| IBIS file k65_180_169wlcsp_derated.ibs generated by Daphne version: 2015.01.22
[IBIS Ver]   4.2
[Comment Char]   |_char
[File Name]   k65_180_169wlcsp_derated.ibs
[File Rev]   1.0
[Date]   Mon Feb  9 00:49:59 2015
[Source]   FSL Viper 2015.01.22
[Notes]
[Disclaimer] IMPORTANT NOTICE
  This information is provided on an AS IS basis and without warranty.
  IN NO EVENT SHALL Freescale BE LIABLE FOR INCIDENTAL OR CONSEQUENTIAL
  DAMAGES ARISING FROM USE OF THIS INFORMATION. THIS DISCLAIMER OF
  WARRANTY EXTENDS TO THE USER OF THE INFORMATION, AND TO THEIR CUSTOMERS
  OR USERS OF PRODUCTS  AND IS IN LIEU OF ALL WARRANTIES WHETHER EXPRESS,
  IMPLIED, OR STATUTORY, INCLUDING IMPLIED WARRANTIES OF MERCHANTABILITY
  OR FITNESS FOR PARTICULAR PURPOSE.
  Freescale does not represent or warrant that the information furnished
  hereunder is free of infringement of any third party patents,
  copyrights, trade secrets, or other intellectual property rights.
  Freescale does not represent or warrant that the information is free of
  defect, or that it meets any particular standard, requirements or need
  of the user of the infomation or their customers.
  Freescale reserves the right to change the information in this file
  without notice.
   http://www.freescale.com
[Copyright]   (C) Copyright Freescale 2004 - 2015, All Rights Reserved.
|   k65_169wlcsp
[Component]   k65_169wlcsp
[Manufacturer]   FREESCALE
[Package]
| variable   typ   min   max
R_pkg   0.15383   6.1113e-3   0.52143
L_pkg   5.764e-10   2.255e-11   1.965e-9
C_pkg   5.451e-13   3.559e-13   3.23e-12
[Pin] signal_name   model_name   R_pin   L_pin   C_pin
A1   PTC4   p_io_fast_hd_84u3v_6m   0.023732  8.85e-11  3.766e-13
A2   PTC9   p_io_fast_84u3v_6m   0.018375  6.862e-11 3.613e-13
A3   PTC13   p_io_fast_84u3v_6m   0.018129  6.765e-11 3.623e-13
A4   PTC15   p_io_fast_84u3v_6m   0.026124  9.752e-11 3.789e-13
A5   PTC16   p_io_fast_84u3v_6m   0.022637  8.435e-11 3.688e-13
A6   PTC24   p_io_fast_84u3v_6m   0.022119  8.262e-11 3.667e-13
A7   PTC27   p_io_fast_84u3v_6m   0.013327  4.926e-11 3.772e-13
A8   PTD1   p_io_fast_84u3v_6m   0.020798  7.767e-11 3.64e-13
A9   PTD5   p_io_fast_hd_84u3v_6m   0.024872  9.264e-11 3.787e-13
A10   PTD7   p_io_fast_hd_84u3v_6m   0.056991  2.143e-10 3.903e-13
A11   PTD10   p_io_fast_84u3v_6m   0.038132  1.422e-10 3.951e-13
A12   PTD13   p_io_fast_84u3v_6m   0.030801  1.148e-10 3.876e-13
A13   PTE1   p_io_fast_84u3v_6m   0.028905  9.982e-11 3.814e-13
B1   PTC3   p_io_fast_hd_84u3v_6m   0.02893   1.024e-10 3.939e-13
B2   PTC5   p_io_fast_84u3v_6m   0.11805   4.455e-10 4.334e-13
B3   PTC10   p_io_fast_84u3v_6m   0.083692  3.154e-10 4.487e-13
B4   PTC14   p_io_fast_84u3v_6m   0.076299  2.875e-10 4.432e-13
B5   PTC17   p_io_fast_84u3v_6m   0.081732  3.078e-10 4.521e-13
B6   PTC19   p_io_fast_84u3v_6m   0.07776   2.928e-10 4.431e-13
B7   PTC28   p_io_fast_84u3v_6m   0.095167  3.59e-10  4.232e-13
B8   PTD2   p_io_fast_84u3v_6m   0.098354  3.71e-10  4.199e-13
B9   PTD6   p_io_fast_hd_84u3v_6m   0.11099   4.135e-10 4.308e-13
B10   PTD9   p_io_fast_84u3v_6m   0.10858   4.097e-10 4.919e-13
B11   PTD14   p_io_fast_84u3v_6m   0.15851   5.985e-10 4.673e-13
B12   PTE2   p_io_fast_84u3v_6m   0.093952  3.43e-10  4.731e-13
B13   PTE3   p_io_fast_84u3v_6m   0.040384  1.405e-10 4.018e-13
C1   PTC0   p_io_fast_84u3v_6m   0.045045  1.537e-10 3.845e-13
C2   PTC1   p_io_fast_84u3v_6m   0.09143   3.347e-10 4.691e-13
C3   PTC6   p_io_fast_84u3v_6m   0.21207   8.018e-10 5.038e-13
C4   PTC8   p_io_fast_84u3v_6m   0.24924   9.43e-10  5.323e-13
C5   PTC12   p_io_fast_84u3v_6m   0.19362   7.319e-10 6.054e-13
C6   PTC18   p_io_fast_84u3v_6m   0.13228   4.993e-10 5.174e-13
C7   PTC29   p_io_fast_84u3v_6m   0.17049   6.443e-10 4.713e-13
C8   PTD3   p_io_fast_84u3v_6m   0.1722   6.501e-10 4.686e-13
C9   PTD8   p_io_fast_84u3v_6m   0.18018   6.805e-10 5.792e-13
C10   PTD12   p_io_fast_84u3v_6m   0.23589   8.918e-10 5.241e-13
C11   PTE0   p_io_fast_84u3v_6m   0.18527   6.998e-10 5.94e-13
C12   PTE4   p_io_fast_84u3v_6m   0.085377  3.141e-10 4.617e-13
C13   PTE6   p_io_fast_84u3v_6m   0.024732  8.58e-11  3.806e-13
D1   PTB21   p_io_fast_84u3v_6m   0.042455  1.491e-10 4.054e-13
D2   PTB22   p_io_fast_84u3v_6m   0.095598  3.503e-10 4.76e-13
D3   PTB23   p_io_fast_84u3v_6m   0.15005   5.554e-10 5.454e-13
D4   PTC2   p_io_fast_84u3v_6m   0.22558   8.431e-10 6.474e-13
D5   PTC7   p_io_fast_84u3v_6m   0.36302   1.373e-9  6.151e-13
D6   PTC11   p_io_fast_84u3v_6m   0.28083   1.062e-9  7.192e-13
D7   PTC25   p_io_fast_84u3v_6m   0.24737   9.352e-10 5.244e-13
D8   PTD0   p_io_fast_84u3v_6m   0.24069   9.1e-10   5.199e-13
D9   PTD11   p_io_fast_84u3v_6m   0.32905   1.244e-9  5.966e-13
D10   PTD15   p_io_fast_84u3v_6m   0.25457   9.624e-10 6.869e-13
D11   PTE5   p_io_fast_84u3v_6m   0.1582   5.936e-10 5.659e-13
D12   PTE8   p_io_fast_84u3v_6m   0.080106  2.969e-10 4.574e-13
D13   PTE9   p_io_fast_84u3v_6m   0.02551   8.823e-11 3.825e-13
E1   PTB16   p_io_fast_84u3v_6m   0.039133  1.335e-10 6.001e-13
E2   PTB17   p_io_fast_84u3v_6m   0.11944   4.359e-10 4.4e-13
E3   PTB18   p_io_fast_84u3v_6m   0.19455   7.186e-10 4.928e-13
E4   PTB19   p_io_fast_84u3v_6m   0.27322   1.019e-9  5.501e-13
E5   PTB20   p_io_fast_84u3v_6m   0.35239   1.319e-9  6.063e-13
E6   VDD   POWER   NA   NA   NA
E7   VDD   POWER   NA   NA   NA
E8   PTC26   p_io_fast_84u3v_6m   0.3454   1.307e-9  5.975e-13
E9   VDD   POWER   NA   NA   NA
E10   PTE7   p_io_fast_84u3v_6m   0.21217   7.942e-10 6.304e-13
E11   PTE11   p_io_fast_84u3v_6m   0.13874   5.131e-10 5.227e-13
E12   PTE12   p_io_fast_84u3v_6m   0.081914  3.035e-10 4.562e-13
E13   VDD   POWER   NA   NA   NA
F1   PTB15   p_io_fast_84u3v_6m   0.037248  1.296e-10 5.892e-13
F2   PTB14   p_io_fast_84u3v_6m   0.1199   4.397e-10 4.397e-13
F3   PTB13   p_io_fast_84u3v_6m   0.18578   6.906e-10 4.872e-13
F4   PTB12   p_io_fast_84u3v_6m   0.25216   9.457e-10 5.394e-13
F5   PTB11   p_io_fast_84u3v_6m   0.31655   1.193e-9  5.865e-13
F6   VSS   GND   NA   NA   NA
F7   VSS   GND   NA   NA   NA
F8   PTD4   p_io_fast_hd_84u3v_6m   0.38395   1.452e-9  6.24e-13
F9   VDD   POWER   NA   NA   NA
F10   PTE10   p_io_fast_84u3v_6m   0.23213   8.667e-10 6.526e-13
F11   PTE17   p_io_fast_84u3v_6m   0.18215   6.744e-10 4.906e-13
F12   PTE19   p_io_fast_84u3v_6m   0.12637   4.625e-10 4.553e-13
F13   VSS   GND   NA   NA   NA
G1   PTB10   p_io_fast_84u3v_6m   0.025215  8.729e-11 3.82e-13
G2   PTB9   p_io_fast_84u3v_6m   0.11037   3.994e-10 4.374e-13
G3   PTB8   p_io_fast_84u3v_6m   0.17439   6.504e-10 4.747e-13
G4   PTB7   p_io_fast_84u3v_6m   0.24603   9.208e-10 5.301e-13
G5   PTB6   p_io_fast_84u3v_6m   0.32096   1.199e-9  5.843e-13
G6   VDD   POWER   NA   NA   NA
G7   VSS   GND   NA   NA   NA
G8   VSS   GND   NA   NA   NA
G9   PTE16   p_io_fast_84u3v_6m   0.36509   1.369e-9  6.196e-13
G10   PTE18   p_io_fast_84u3v_6m   0.28872   1.074e-9  5.683e-13
G11   VREGOUT   POWER   0.28285   1.07e-9   6.103e-13
G12   VREGIN0   POWER   0.11913   4.476e-10 5.637e-13
G13   USB0DP   NC   0.040105  1.411e-10 4.143e-13
H1   PTB5   p_io_fast_84u3v_6m   0.02475   8.564e-11 3.808e-13
H2   PTB4   p_io_fast_84u3v_6m   0.082285  3.039e-10 4.551e-13
H3   PTB3   p_io_fast_84u3v_6m   0.1553   5.764e-10 5.545e-13
H4   PTB0   p_io_fast_hd_84u3v_6m   0.22249   8.274e-10 6.597e-13
H5   PTA31   p_io_fast_84u3v_6m   0.28767   1.078e-9  7.367e-13
H6   VSS   GND   NA   NA   NA
H7   VSS   GND   NA   NA   NA
H8   TAMPER6   p_io_84u3v_6m   0.40121   1.518e-9  6.321e-13
H9   TAMPER2   p_io_84u3v_6m   0.42606   1.613e-9  6.532e-13
H10   TAMPER1   p_io_84u3v_6m   0.43051   1.629e-9  6.596e-13
H11   ADC1SE16_CMP2IN2_ADC0SE22   NC   0.52143   1.965e-9  7.296e-13
H12   VREGIN1   POWER   0.081939  3.085e-10 5.05e-13
H13   USB0DM   NC   0.042727  1.498e-10 4.137e-13
J1   PTB2   p_io_fast_84u3v_6m   0.036541  1.276e-10 3.982e-13
J2   PTB1   p_io_fast_hd_84u3v_6m   0.090111  3.314e-10 6.961e-13
J3   PTA26   p_io_fast_84u3v_6m   0.30189   1.127e-9  5.72e-13
J4   PTA25   p_io_fast_84u3v_6m   0.36496   1.363e-9  6.172e-13
J5   PTA9   p_io_fast_84u3v_6m   0.36508   1.381e-9  6.152e-13
J6   PTA3   p_io_fast_84u3v_6m   0.31893   1.206e-9  5.775e-13
J7   PTE27   p_io_fast_84u3v_6m   0.30618   1.158e-9  5.656e-13
J8   TAMPER7   p_io_84u3v_6m   0.32279   1.223e-9  5.759e-13
J9   TAMPER3   p_io_84u3v_6m   0.34626   1.31e-9   5.974e-13
J10   TAMPER0_RTCWAKEUP   p_io_84u3v_6m   0.37467   1.418e-9  6.188e-13
J11   ADC1DP1   NC   0.18235   6.796e-10 6.053e-13
J12   USB1VSS   GND   NA   NA   NA
J13   USB1DP   NC   0.035762  1.286e-10 4.048e-13
K1   PTA30   p_io_fast_84u3v_6m   0.044808  1.573e-10 4.101e-13
K2   PTA29   p_io_fast_84u3v_6m   0.097255  3.561e-10 4.771e-13
K3   PTA24   p_io_fast_84u3v_6m   0.26349   9.776e-10 5.455e-13
K4   PTA16   p_io_fast_84u3v_6m   0.28673   1.085e-9  5.539e-13
K5   PTA10   p_io_fast_84u3v_6m   0.30667   1.16e-9   5.738e-13
K6   PTA4   p_io_flt_84u3v_6m   0.2545   9.6e-10   5.382e-13
K7   PTE28   p_io_fast_84u3v_6m   0.24086   9.108e-10 5.207e-13
K8   VDD   POWER   NA   NA   NA
K9   TAMPER5   p_io_84u3v_6m   0.19261   7.28e-10  6.086e-13
K10   ADC0SE16_CMP1IN2_ADC0SE21   NC   0.35901   1.358e-9  6.097e-13
K11   ADC1DM1   NC   0.18943   7.059e-10 6.096e-13
K12   USB1VBUS   POWER   0.079962  2.996e-10 5.011e-13
K13   USB1DM   NC   0.033877  1.207e-10 4.021e-13
L1   PTA28   p_io_fast_84u3v_6m   0.032314  1.102e-10 3.958e-13
L2   PTA27   p_io_fast_84u3v_6m   0.11465   4.175e-10 4.36e-13
L3   PTA17   p_io_fast_84u3v_6m   0.2195   8.299e-10 5.116e-13
L4   PTA15   p_io_fast_84u3v_6m   0.20307   7.686e-10 5.042e-13
L5   PTA13   p_io_fast_84u3v_6m   0.17543   6.626e-10 5.788e-13
L6   PTA7   p_io_fast_84u3v_6m   0.20442   7.727e-10 4.991e-13
L7   PTA2   p_io_fast_84u3v_6m   0.17109   6.464e-10 4.707e-13
L8   PTE26   p_io_fast_84u3v_6m   0.16532   6.25e-10  4.717e-13
L9   VBAT   POWER   0.19977   7.554e-10 4.914e-13
L10   VREFOUT_CMP1IN5_CMP0IN5_ADC1SE18   NC   0.27856   1.053e-9  5.522e-13
L11   VDDA   POWER   0.17063   6.391e-10 5.765e-13
L12   ADC1DP0_ADC0DP3   NC   0.16003   5.889e-10 4.807e-13
L13   ADC0DP0_ADC1DP3   NC   0.037046  1.324e-10 4.003e-13
M1   RESETB   p_io_84u3v_6m   0.019078  6.944e-11 5.589e-13
M2   VSS   GND   NA   NA   NA
M3   VDD   POWER   NA   NA   NA
M4   PTA12   p_io_fast_84u3v_6m   0.081486  3.07e-10  4.542e-13
M5   PTA8   p_io_fast_84u3v_6m   0.11651   4.399e-10 4.289e-13
M6   VDD   POWER   NA   NA   NA
M7   PTA1   p_io_fast_84u3v_6m   0.098968  3.734e-10 4.207e-13
M8   PTE25   p_io_fast_84u3v_6m   0.095813  3.628e-10 4.167e-13
M9   XTAL32   NC   0.088546  3.341e-10 4.617e-13
M10   DAC0OUT_CMP1IN3_ADC0SE23   NC   0.20614   7.807e-10 4.99e-13
M11   VREFH   POWER   0.18763   6.924e-10 4.814e-13
M12   ADC1DM0_ADC0DM3   NC   0.15794   5.866e-10 4.751e-13
M13   ADC0DM0_ADC1DM3   NC   0.039342  1.372e-10 3.982e-13
N1   PTA18   p_io_fast_84u3v_6m   0.022116  8.299e-11 3.67e-13
N2   PTA19   p_io_fast_84u3v_6m   0.11411   4.319e-10 4.97e-13
N3   PTA14   p_io_fast_84u3v_6m   0.021852  8.118e-11 3.749e-13
N4   PTA11   p_io_fast_84u3v_6m   0.031632  1.18e-10  3.886e-13
N5   PTA6   p_io_fast_84u3v_6m   0.024938  9.306e-11 3.793e-13
N6   PTA5   p_io_fast_84u3v_6m   0.024667  9.198e-11 3.788e-13
N7   PTA0   p_io_fast_84u3v_6m   0.022655  8.503e-11 3.669e-13
N8   PTE24   p_io_fast_84u3v_6m   0.021201  8.018e-11 3.559e-13
N9   EXTAL32   NC   0.03501   1.309e-10 3.905e-13
N10   TAMPER4   p_io_84u3v_6m   0.026057  9.759e-11 3.763e-13
N11   DAC1OUT_CMP0IN4_CMP2IN3_ADC1SE23   NC   0.081432  2.74e-10  4.161e-13
N12   VREFL   NC   0.11001   4.012e-10 4.432e-13
N13   VSSA   GND   0.025288  8.758e-11 3.839e-13
[Pin Mapping]   pulldown_ref   pullup_ref
A1   NC   NC
A2   NC   NC
A3   NC   NC
A4   NC   NC
A5   NC   NC
A6   NC   NC
A7   NC   NC
A8   NC   NC
A9   NC   NC
A10   NC   NC
A11   NC   NC
A12   NC   NC
A13   NC   NC
B1   NC   NC
B2   NC   NC
B3   NC   NC
B4   NC   NC
B5   NC   NC
B6   NC   NC
B7   NC   NC
B8   NC   NC
B9   NC   NC
B10   NC   NC
B11   NC   NC
B12   NC   NC
B13   NC   NC
C1   NC   NC
C2   NC   NC
C3   NC   NC
C4   NC   NC
C5   NC   NC
C6   NC   NC
C7   NC   NC
C8   NC   NC
C9   NC   NC
C10   NC   NC
C11   NC   NC
C12   NC   NC
C13   NC   NC
D1   NC   NC
D2   NC   NC
D3   NC   NC
D4   NC   NC
D5   NC   NC
D6   NC   NC
D7   NC   NC
D8   NC   NC
D9   NC   NC
D10   NC   NC
D11   NC   NC
D12   NC   NC
D13   NC   NC
E1   NC   NC
E2   NC   NC
E3   NC   NC
E4   NC   NC
E5   NC   NC
E6   NC   VDD
E7   NC   VDD
E8   NC   NC
E9   NC   VDD
E10   NC   NC
E11   NC   NC
E12   NC   NC
E13   NC   VDD
F1   NC   NC
F2   NC   NC
F3   NC   NC
F4   NC   NC
F5   NC   NC
F6   VSS   NC
F7   VSS   NC
F8   NC   NC
F9   NC   VDD
F10   NC   NC
F11   NC   NC
F12   NC   NC
F13   VSS   NC
G1   NC   NC
G2   NC   NC
G3   NC   NC
G4   NC   NC
G5   NC   NC
G6   NC   VDD
G7   VSS   NC
G8   VSS   NC
G9   NC   NC
G10   NC   NC
G11   NC   VREGOUT
G12   NC   VREGIN0
G13   NC   NC
H1   NC   NC
H2   NC   NC
H3   NC   NC
H4   NC   NC
H5   NC   NC
H6   VSS   NC
H7   VSS   NC
H8   NC   NC
H9   NC   NC
H10   NC   NC
H11   NC   NC
H12   NC   VREGIN1
H13   NC   NC
J1   NC   NC
J2   NC   NC
J3   NC   NC
J4   NC   NC
J5   NC   NC
J6   NC   NC
J7   NC   NC
J8   NC   NC
J9   NC   NC
J10   NC   NC
J11   NC   NC
J12   USB1VSS   NC
J13   NC   NC
K1   NC   NC
K2   NC   NC
K3   NC   NC
K4   NC   NC
K5   NC   NC
K6   NC   NC
K7   NC   NC
K8   NC   VDD
K9   NC   NC
K10   NC   NC
K11   NC   NC
K12   NC   USB1VBUS
K13   NC   NC
L1   NC   NC
L2   NC   NC
L3   NC   NC
L4   NC   NC
L5   NC   NC
L6   NC   NC
L7   NC   NC
L8   NC   NC
L9   NC   VBAT
L10   NC   NC
L11   NC   VDDA
L12   NC   NC
L13   NC   NC
M1   NC   NC
M2   VSS   NC
M3   NC   VDD
M4   NC   NC
M5   NC   NC
M6   NC   VDD
M7   NC   NC
M8   NC   NC
M9   NC   NC
M10   NC   NC
M11   NC   VREFH
M12   NC   NC
M13   NC   NC
N1   NC   NC
N2   NC   NC
N3   NC   NC
N4   NC   NC
N5   NC   NC
N6   NC   NC
N7   NC   NC
N8   NC   NC
N9   NC   NC
N10   NC   NC
N11   NC   NC
N12   NC   NC
N13   VSSA   NC
|*   Model Selector   *
[Model Selector] p_io_84u3v_6m
p_io_84u3v_6m_sre0   io, without slew rate
p_io_84u3v_6m_sre1   io, with slew rate
[Model Selector] p_io_fast_84u3v_6m
p_io_fast_84u3v_6m_sre0   io, without slew rate
p_io_fast_84u3v_6m_sre1   io, with slew rate
[Model Selector] p_io_fast_hd_84u3v_6m
p_io_fast_hd_84u3v_6m_obe1dse0sre0   io 5mA, without slew rate
p_io_fast_hd_84u3v_6m_obe1dse0sre1   io 5mA, with slew rate
p_io_fast_hd_84u3v_6m_obe1dse1sre0   io 20mA, without slew rate
p_io_fast_hd_84u3v_6m_obe1dse1sre1   io 20mA, with slew rate
[Model Selector] p_io_flt_84u3v_6m
p_io_flt_84u3v_6m_sre0   io_flt, without slew rate
p_io_flt_84u3v_6m_sre1   io_flt, with slew rate
| End [Component] k65_169wlcsp
| Models and submodels in the file (10): p_io_84u3v_6m_sre0 (I/O), p_io_84u3v_6m_sre1 (I/O), p_io_fast_84u3v_6m_sre0 (I/O), p_io_fast_84u3v_6m_sre1 (I/O), p_io_fast_hd_84u3v_6m_obe1dse0sre0 (I/O), p_io_fast_hd_84u3v_6m_obe1dse0sre1 (I/O), p_io_fast_hd_84u3v_6m_obe1dse1sre0 (I/O), p_io_fast_hd_84u3v_6m_obe1dse1sre1 (I/O), p_io_flt_84u3v_6m_sre0 (I/O), p_io_flt_84u3v_6m_sre1 (I/O)
